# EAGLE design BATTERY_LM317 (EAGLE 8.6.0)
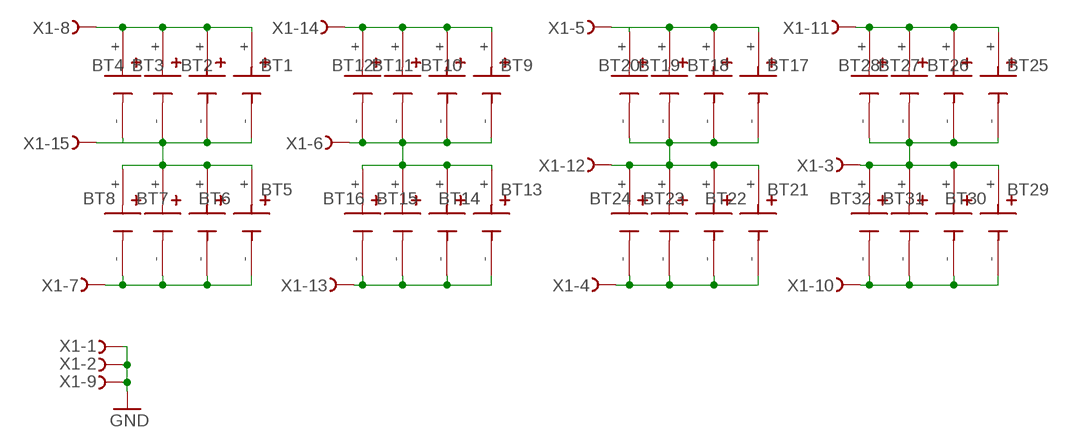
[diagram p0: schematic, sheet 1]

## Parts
BT1  BHDL  [BAT_BHDL]
BT2  BHCL  [BAT_BHCL]
BT3  BCAAL  [BAT_BCAAL]
BT4  BCAAAL  [BAT_BCAAAL]
BT5  BHDL  [BAT_BHDL]
BT6  BHCL  [BAT_BHCL]
BT7  BCAAL  [BAT_BCAAL]
BT8  BCAAAL  [BAT_BCAAAL]
BT9  BHDL  [BAT_BHDL]
BT10  BHCL  [BAT_BHCL]
BT11  BCAAL  [BAT_BCAAL]
BT12  BCAAAL  [BAT_BCAAAL]
BT13  BHDL  [BAT_BHDL]
BT14  BHCL  [BAT_BHCL]
BT15  BCAAL  [BAT_BCAAL]
BT16  BCAAAL  [BAT_BCAAAL]
BT17  BHDL  [BAT_BHDL]
BT18  BHCL  [BAT_BHCL]
BT19  BCAAL  [BAT_BCAAL]
BT20  BCAAAL  [BAT_BCAAAL]
BT21  BHDL  [BAT_BHDL]
BT22  BHCL  [BAT_BHCL]
BT23  BCAAL  [BAT_BCAAL]
BT24  BCAAAL  [BAT_BCAAAL]
BT25  BHDL  [BAT_BHDL]
BT26  BHCL  [BAT_BHCL]
BT27  BCAAL  [BAT_BCAAL]
BT28  BCAAAL  [BAT_BCAAAL]
BT29  BHDL  [BAT_BHDL]
BT30  BHCL  [BAT_BHCL]
BT31  BCAAL  [BAT_BCAAL]
BT32  BCAAAL  [BAT_BCAAAL]
X1  F15.590S  [177-015-212-FEMALE]

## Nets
GND: X1.1 X1.2 X1.9
N$1: BT1.+ BT2.+ BT3.+ BT4.+ X1.8
N$2: BT1.- BT2.- BT3.- BT4.- BT5.+ BT6.+ BT7.+ BT8.+ X1.15
N$3: BT9.+ BT10.+ BT11.+ BT12.+ X1.14
N$4: BT5.- BT6.- BT7.- BT8.- X1.7
N$5: BT9.- BT10.- BT11.- BT12.- BT13.+ BT14.+ BT15.+ BT16.+ X1.6
N$6: BT13.- BT14.- BT15.- BT16.- X1.13
N$7: BT17.+ BT18.+ BT19.+ BT20.+ X1.5
N$8: BT17.- BT18.- BT19.- BT20.- BT21.+ BT22.+ BT23.+ BT24.+ X1.12
N$9: BT21.- BT22.- BT23.- BT24.- X1.4
N$10: BT25.+ BT26.+ BT27.+ BT28.+ X1.11
N$11: BT25.- BT26.- BT27.- BT28.- BT29.+ BT30.+ BT31.+ BT32.+ X1.3
N$12: BT29.- BT30.- BT31.- BT32.- X1.10

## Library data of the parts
BT1 BT5 BT9 BT13 BT17 BT21 BT25 BT29 = BHDL D CELL:BHDL: Battery Holder (Open) D 1 Cell Solder Lug Check availability; AVAILABILITY: In Stock; CHECK_PRICES: https://www.snapeda.com/parts/BHDL/Memory+Protection+Devices/view-part/?ref=eda; DESCRIPTION: Battery Holder 1 Cells D Size Polypropylene; MF: MPD (Memory Protection Devices); MP: BHDL; PACKAGE: None; PRICE: None; SNAPEDA_LINK: https://www.snapeda.com/parts/BHDL/Memory+Protection+Devices/view-part/?ref=snap
BT2 BT6 BT10 BT14 BT18 BT22 BT26 BT30 = BHCL C CELL:BHCL: Battery Holder (Open) C 1 Cell Solder Lug Check availability; AVAILABILITY: In Stock; CHECK_PRICES: https://www.snapeda.com/parts/BHCL/Memory+Protection+Devices/view-part/?ref=eda; DESCRIPTION: Battery Holder (Open) C 1 Cell Solder Lug; MF: MPD (Memory Protection Devices); MP: BHCL; PACKAGE: None; PRICE: None; SNAPEDA_LINK: https://www.snapeda.com/parts/BHCL/Memory+Protection+Devices/view-part/?ref=snap
BT3 BT7 BT11 BT15 BT19 BT23 BT27 BT31 = BCAAL:BCAAL: AA Battery Holder Check availability; AVAILABILITY: In Stock; CHECK_PRICES: https://www.snapeda.com/parts/BCAAL/Memory+Protection+Devices/view-part/?ref=eda; DESCRIPTION: Battery Holder (Open) AA 1 Cell Solder Lug; MF: MPD (Memory Protection Devices); MP: BCAAL; PACKAGE: None; PRICE: None; SNAPEDA_LINK: https://www.snapeda.com/parts/BCAAL/Memory+Protection+Devices/view-part/?ref=snap
BT4 BT8 BT12 BT16 BT20 BT24 BT28 BT32 = BCAAAL:BCAAAL: AAA Battery Holder Check availability; AVAILABILITY: Not in stock; CHECK_PRICES: https://www.snapeda.com/parts/BCAAAL/Memory+Protection+Devices/view-part/?ref=eda; DESCRIPTION: Battery Holder (Open) AAA 1 Cell Solder Lug; MF: Memory Protection Dev.; MP: BCAAAL; PACKAGE: None; PRICE: None; SNAPEDA_LINK: https://www.snapeda.com/parts/BCAAAL/Memory+Protection+Devices/view-part/?ref=snap
X1 = con-subd:F15?S: SUB-D; OC_FARNELL: unknown; OC_NEWARK: unknown

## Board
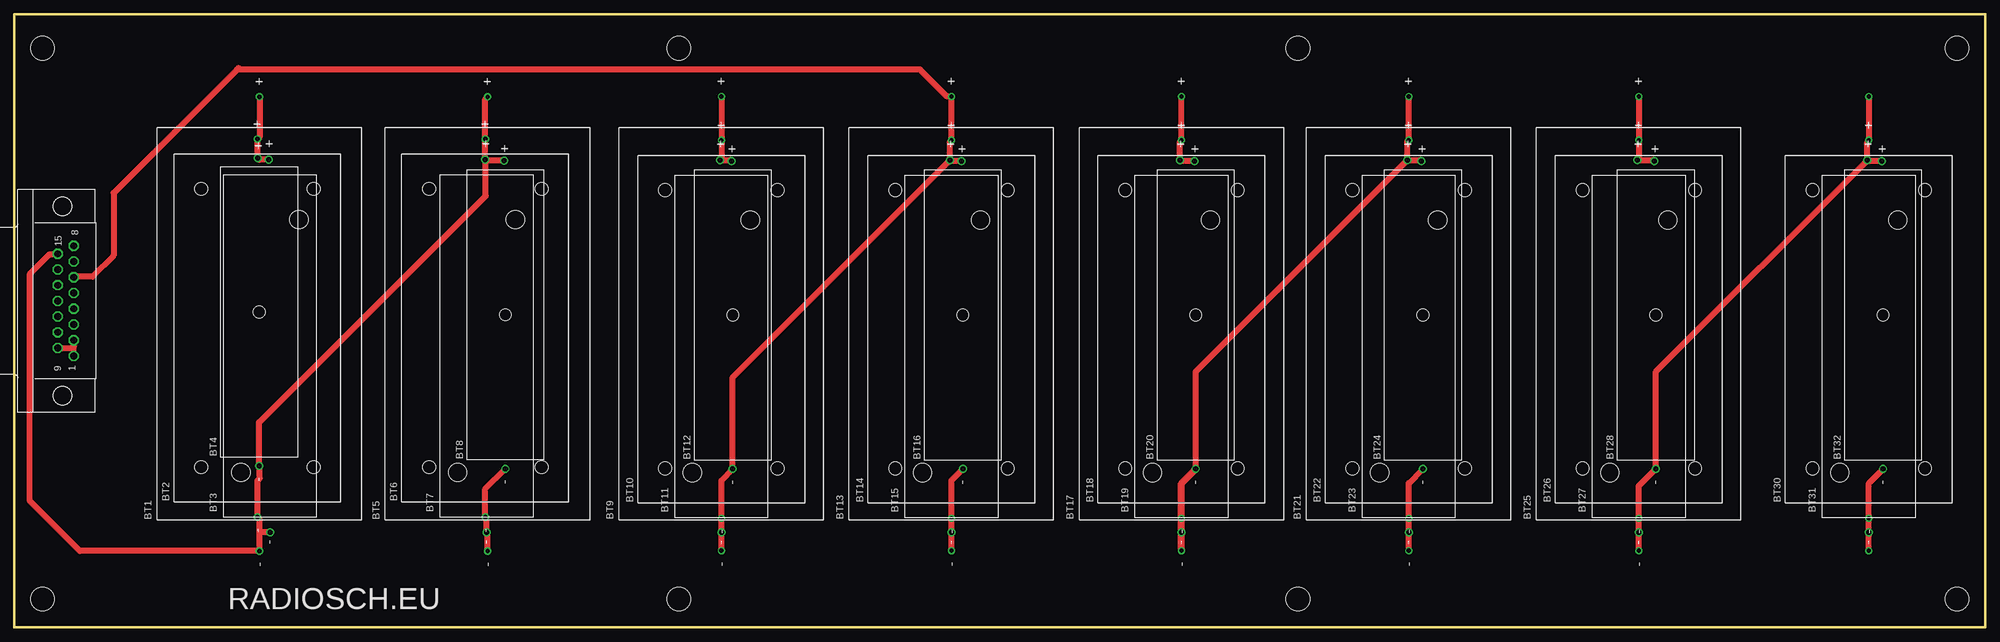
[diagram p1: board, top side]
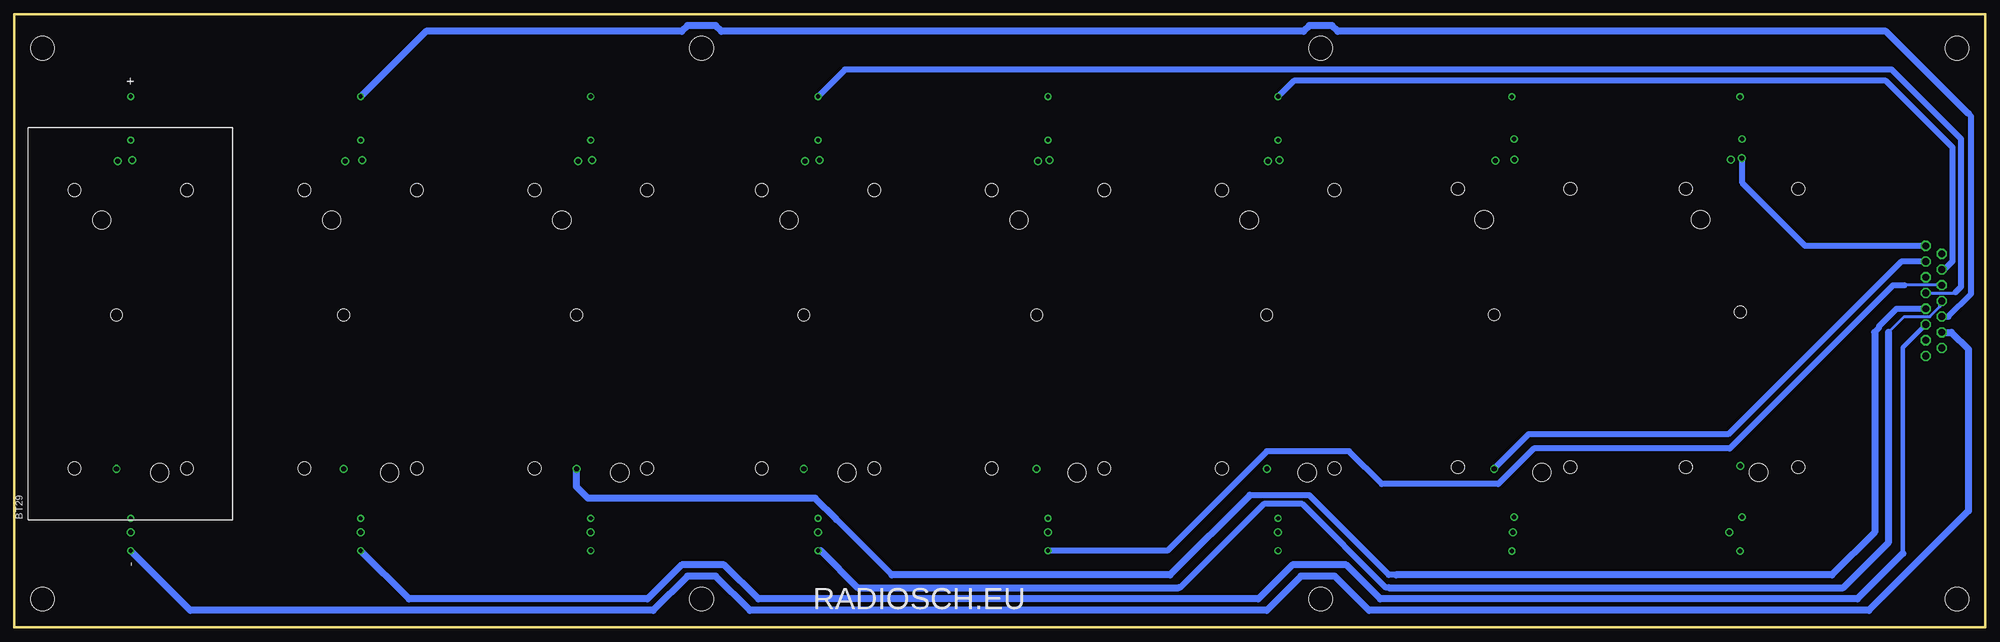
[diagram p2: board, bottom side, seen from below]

Size 347 x 108 mm. Coordinates in mm from the lower left corner, seen from the top.
Outline: 0,0 347,0 347,108 0,108 0,0
Copper layers (1*16): Top 0.035mm / dielectric 1.5mm / Bottom 0.035mm
Design rules "default": minimum track width 10mil, minimum drill 24mil, track to track 8mil, track to pad 8mil, pad to pad 8mil, via to via 8mil, smd to smd 8mil, copper to edge 40mil, drill to drill 8mil, minimum pad ring 10mil, minimum via ring 8mil, stop-mask expansion 4mil, vias tented up to drill 0mil, thermal gap 10mil
Holes 4.2 mm at 5,5 342,5 117,5 226,5 5,102 342,102 117,102 226,102

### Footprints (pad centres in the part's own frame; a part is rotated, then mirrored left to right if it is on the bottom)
BAT_BHDL = drill 0.755: + 40,0; - -40,0
BAT_BHCL = drill 0.755: + 33.3,0; - -33.3,0 | hole 2.28: -24.5,9.905; 24.5,9.905; -24.5,-9.905; 24.5,-9.905
BAT_BCAAL = drill 0.89: + 32.8,0.24; - -32.8,0 | hole 3.25: 22.25,-5.1; -22.25,5.1
BAT_BCAAAL = drill 0.89: + 27.12,0.24; - -27.12,0 | hole 2.11: 0,0
177-015-212-FEMALE = drill 1.194 pad 1.524 octagon: 1 -9.69,-1.99; 2 -6.921,-1.99; 3 -4.153,-1.99; 4 -1.384,-1.99; 5 1.384,-1.99; 6 4.153,-1.99; 7 6.921,-1.99; 8 9.69,-1.99; 9 -8.306,0.854; 10 -5.537,0.854; 11 -2.769,0.854; 12 0,0.854; 13 2.769,0.854; 14 5.537,0.854; 15 8.306,0.854

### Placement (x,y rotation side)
BT1  43.18,53.45 90 top
BT2  42.82,52.72 90 top
BT3  45.03,49.56 90 top
BT4  43.12,55.56 90 top
BT5  83.34,53.45 90 top
BT6  82.94,52.72 90 top
BT7  83.15,49.56 90 top
BT8  86.47,55.06 90 top
BT9  124.5,53.5 90 top
BT10  124.5,52.5 90 top
BT11  124.5,49.5 90 top
BT12  126.5,55 90 top
BT13  165,53.5 90 top
BT14  165,52.5 90 top
BT15  165,49.5 90 top
BT16  167,55 90 top
BT17  205.5,53.5 90 top
BT18  205.5,52.5 90 top
BT19  205.5,49.5 90 top
BT20  208,55 90 top
BT21  245.5,53.5 90 top
BT22  245.5,52.5 90 top
BT23  245.5,49.5 90 top
BT24  248,55 90 top
BT25  286,53.5 90 top
BT26  286,52.5 90 top
BT27  286,49.5 90 top
BT28  289,55 90 top
BT29  326.5,53.5 90 bottom
BT30  326.5,52.5 90 top
BT31  326.5,49.5 90 top
BT32  329,55 90 top
X1  8.5,57.5 90 top

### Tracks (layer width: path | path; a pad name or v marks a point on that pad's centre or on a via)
GND
  Top 1.016: X1.1 10.49,49.5 | 10.49,49.5 X1.2 | X1.9 10.18,49.19 10.49,49.5
N$1
  Top 1.016: BT1.+ 43.18,86.38 BT2.+ 42.88,85.96 BT4.+ 43.2,82.36 BT3.+
  Bottom 1.016: X1.8 31.69,67.19 42.75,78.25 42.75,82.55 BT4.+
N$2
  Top 1.016: X1.15 7.59,65.75 6.25,65.75 2.75,62.25 2.75,22.25 11.55,13.45 BT1.- 43.18,17 | 83,82.27 83,76 43.12,36.12 BT4.- 43.25,28.31 43.25,26.25 42.82,25.82 BT2.- 43.18,19.06 43.18,17 | 83,82.27 BT7.+ 82.91,85.99 BT6.+ 82.94,93.05 BT5.+ | 83,82.27 86.14,82.27 BT8.+ | BT3.- 43.76,16.76 43.75,16.75 43.43,16.75 43.18,17
N$3
  Top 1.016: BT9.+ BT10.+ 124.5,82.54 BT11.+ 126.08,82.3 BT12.+
  Bottom 1.016: BT9.+ 121.75,96.25 17.5,96.25 5.75,84.5 5.75,64.5 7.21,63.04 X1.14
N$4
  Top 1.016: BT5.- 83.34,16.57 BT7.- 83.15,19.21 BT6.- 82.94,24.41 BT8.-
  Bottom 1.016: X1.7 14.83,64.42 45.25,34 80.41,34 BT8.-
N$5
  Top 1.016: 39.5,98.5 39.25,98.25 | 39.25,98.25 17.5,76.5 17.5,65.5 13.75,61.75 10.59,61.75 X1.6 | BT15.+ 126.5,44.04 BT12.- 124.5,25.88 BT10.- BT11.- BT9.- | BT16.+ 164.94,82.12 BT15.+ | BT15.+ 164.76,85.56 BT14.+ BT13.+ 164.25,93.5 159.5,98.25 39.25,98.25
N$6
  Top 1.016: BT13.- BT15.- BT14.- 165,25.88 BT16.-
  Bottom 0.5: X1.13 14.23,60.27 14.25,60.25
  Bottom 1.016: BT13.- 144,13.5 126.5,31 112,31 106.25,25.25 85.75,25.25 79.5,31.5 45,31.5 16.25,60.25 14.25,60.25
N$7
  Top 1.016: BT20.+ 205.44,82.12 BT19.+ 205.26,85.56 BT18.+ BT17.+
  Bottom 0.5: X1.5 5.37,58.88 5.25,59
  Bottom 1.016: BT17.+ 200.75,98.25 16.5,98.25 4.25,86 4.25,60 5.25,59
N$8
  Top 1.016: BT20.- 208,45.04 BT23.+ | BT23.+ 247.58,82.3 BT24.+ | BT23.+ 245.26,85.56 BT22.+ BT21.+
  Top 1.27: BT17.- BT19.- BT18.- 205.5,25.38 BT20.-
  Bottom 0.5: X1.12 8,57.15 8,56.5 9.75,54.75 14.25,54.75 17,52
  Bottom 1.016: 105,7 105.5,7 120.25,21.75 127,21.75 141.75,7 142,7
  Bottom 1.27: BT17.- 205,13.5 198.5,7 142,7 | 105,7 25,7 17,15 17,52
N$9
  Top 1.016: BT24.- 245.5,25.38 BT22.- BT23.- BT21.-
  Bottom 1.016: X1.4 15.63,56.12 18.75,53 18.75,52.75 19.5,52 | 103.75,9.25 105,9.25 119,23.25 129.5,23.25 | 202.25,19 192.5,9.25
  Bottom 1.27: 19.5,52 19.5,16.75 27,9.25 103.75,9.25 | 129.5,23.25 143.5,9.25 192.5,9.25 | 202.25,19 206,22.75 246,22.75 248,24.75 BT24.-
N$10
  Top 1.016: BT25.+ BT26.+ 286,82.54 BT27.+ 288.58,82.3 BT28.+
  Bottom 1.016: X1.11 6.52,54.73 2.5,58.75 2.5,90 3.75,91.25
  Bottom 1.27: 3,90.5 3.75,91.25 17.5,105 114,105 115,106 119,106 120,105 222.5,105 223.5,106 228.5,106 229.5,105 274.5,105 BT25.+
N$11
  Top 1.016: BT25.- BT27.- BT26.- 286,24.88 BT28.- 289,45.04 325.86,81.89 326.08,82.12 | 326.08,82.12 BT31.+ 326.26,85.56 BT30.+ BT29.+ | BT32.+ 326.08,82.12
  Bottom 0.813: 14.5,13 14.5,49.34 X1.3
  Bottom 1.27: 14.5,13 22.5,5 106.5,5 112.5,11 122,11 128,5 216,5 222,11 229.5,11 235.5,5 277.5,5 BT25.-
N$12
  Top 1.016: BT29.- BT31.- BT30.- 326.5,25.38 BT32.-
  Bottom 1.27: X1.10 5.96,51.96 3,49 3,20.5 20.5,3 108.5,3 114.5,9 120.5,9 126.5,3 217.5,3 223.5,9 228.5,9 234.5,3 316,3 BT29.-

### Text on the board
tPlace: RADIOSCH.EU
bPlace: RADIOSCH.EU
